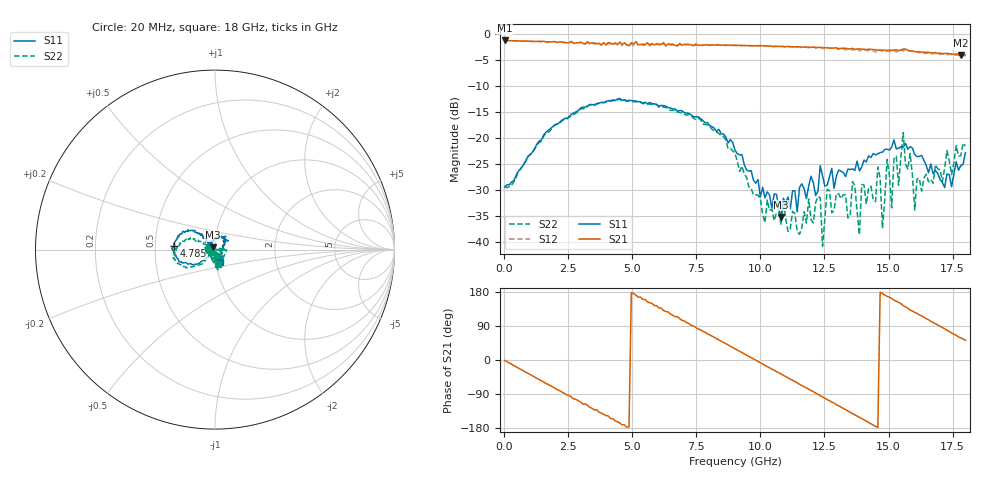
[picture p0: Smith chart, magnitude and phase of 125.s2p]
!Agilent Technologies,N5230A,US43500223,A.07.50.48
!Agilent N5230A: A.07.50.48
!Date: Saturday, January 16, 2016 21:40:08
!Correction: S11(Full 2 Port(1,2))
!S21(Full 2 Port(1,2))
!S12(Full 2 Port(1,2))
!S22(Full 2 Port(1,2))
!S2P File: Measurements: S11, S21, S12, S22:
# Hz S  dB  R 50
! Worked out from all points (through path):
!   201 points, 20 MHz to 18 GHz, reference 50 ohm
!   highest |S21| = -1.16 dB at 20 MHz (marker M1); lowest = -4.0 dB at 17.82 GHz (marker M2)
!   group delay of S21, straight-line fit = 103 ps
!   lowest |S11| = -35.2 dB at 10.81 GHz (marker M3), VSWR 1.04, Z = 48.7 + j1.14 ohm
!   |S11| at or under -10 dB: start of sweep to end of sweep
!   |S22| runs from -40.9 to -12.5 dB; largest |S21 - S12| = 0.077
!   S11 on the Smith chart (normalised r, x): 20 MHz: 0.93, +0.00; 4.785 GHz: 0.63, +0.03; 18 GHz: 1.05, -0.14
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2e7  -29.45 179.0  -1.16 -0.8  -1.17 -0.9  -29.30 177.3
1.5483e9  -19.38 -138.8  -1.30 -58.3  -1.32 -58.7  -19.61 -131.5
3.0766e9  -14.03 -159.3  -1.69 -116.8  -1.63 -116.3  -14.34 -149.9
4.7847e9  -12.81 174.9  -1.97 -177.5  -2.09 179.9  -12.92 -172.3
6.0433e9  -13.83 154.4  -1.84 137.5  -2.06 134.8  -14.04 173.1
7.4817e9  -15.90 140.0  -1.84 85.6  -2.10 83.5  -16.44 157.3
9.01e9  -22.34 130.3  -2.07 29.5  -2.14 26.7  -22.91 154.8
1.0808e10  -35.21 137.6  -2.27 -37.0  -2.34 -40.0  -36.75 -128.2
1.20666e10  -28.61 121.6  -2.45 -83.6  -2.41 -87.4  -36.34 -158.3
1.35949e10  -25.94 111.2  -2.67 -141.2  -3.01 -146.0  -28.39 -118.1
1.38646e10  -26.33 101.4  -2.79 -151.6  -3.19 -156.2  -38.64 -79.2
1.39545e10  -25.56 95.0  -2.84 -154.5  -2.97 -157.5  -28.95 -115.5
1.45838e10  -23.01 78.4  -3.05 -178.0  -2.87 179.5  -25.58 -80.9
1.47636e10  -22.71 68.8  -3.04 175.2  -3.21 172.1  -37.40 -114.6
1.50333e10  -22.30 72.4  -3.02 165.8  -3.32 160.3  -27.09 -124.5
1.51232e10  -21.75 59.6  -3.06 162.2  -3.36 158.2  -33.46 6.5
1.52131e10  -20.35 50.7  -2.97 158.2  -3.14 154.7  -23.94 -42.8
1.53929e10  -21.97 64.3  -3.11 152.0  -3.27 149.4  -29.10 -176.4
1.55727e10  -21.73 37.0  -2.82 143.6  -3.24 141.3  -18.95 -81.8
1.60222e10  -23.16 35.0  -3.29 125.7  -3.46 122.0  -33.88 -56.8
1.78202e10  -25.31 -73.2  -4.00 58.6  -4.25 53.3  -23.40 -63.6
1.8e10  -22.85 -68.0  -3.98 52.0  -4.13 45.8  -21.54 -78.4
